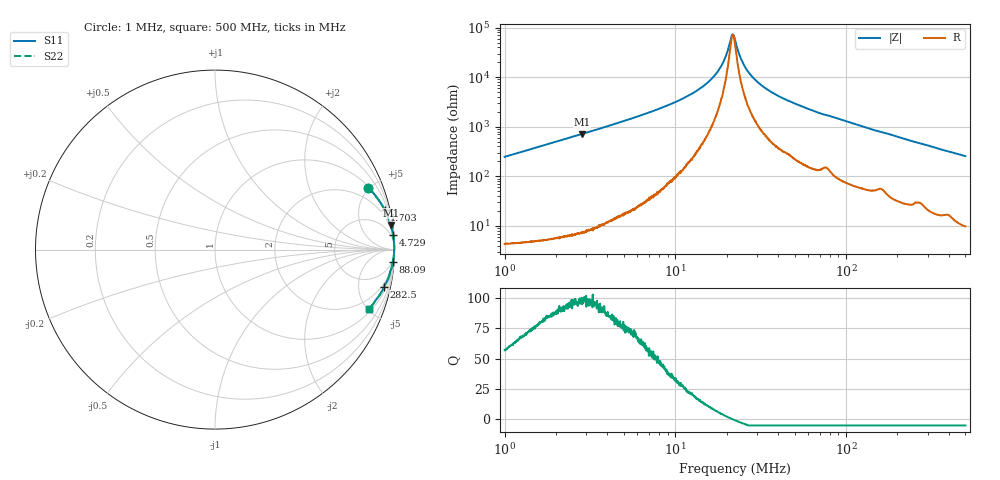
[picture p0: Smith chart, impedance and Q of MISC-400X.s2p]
!s-Parameter Generated by FASTRON Sdn. Bhd.
!FASTRON P/N : MISC-400X
!Keysight Technologies,E4991B,MY54100416,A.01.15
!Date: Thu Mar 26 11:04:12 2026
!Version  : Rev00 Thu Mar 26 11:04:12 2026
!Data & Calibration Information:
!PortZ  Port1:50+j0  Port2:50+j0
!When reading, reference impedance value at option line is always used.
!Remarks : This data is being provided solely for informational purposes.
!Freq	S11	S21	S12	S22
# Hz S dB R 50
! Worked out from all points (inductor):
!   1601 points, 1 MHz to 500 MHz, reference 50 ohm
!   read as one part in series: L = 39.3 uH near 1.032 MHz
!   highest Q = 97.7 at 2.843 MHz (marker M1), where L = 40 uH
!   self-resonance near 21.68 MHz
!   S11 on the Smith chart (normalised r, x): 1 MHz: 1.09, +4.95; 1.703 MHz: 1.10, +8.45; 4.729 MHz: 1, +25; 88.09 MHz: 3, -30; 282.5 MHz: 1.52, -8.95; 500 MHz: 1.20, -5.10
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1000000  -0.71 21.9  -8.57 -67.1  -8.57 -67.1  -0.71 21.9
1702548  -0.26 13.3  -12.78 -76.0  -12.78 -76.0  -0.26 13.3
2820919  -0.10 8.0  -17.10 -81.4  -17.10 -81.4  -0.10 8.0
2842918  -0.10 8.0  -17.17 -81.4  -17.17 -81.4  -0.10 8.0
4728708  -0.04 4.7  -21.81 -84.6  -21.81 -84.6  -0.04 4.7
7957584  -0.02 2.5  -27.16 -86.3  -27.16 -86.3  -0.02 2.5
1.178023e7  -0.01 1.4  -32.35 -86.1  -32.35 -86.1  -0.01 1.4
1.552103e7  -0.01 0.7  -37.93 -84.1  -37.93 -84.1  -0.01 0.7
1.870207e7  -0.01 0.3  -44.84 -77.1  -44.84 -77.1  -0.01 0.3
1.97472e7  -0.01 0.2  -48.48 -69.3  -48.48 -69.3  -0.01 0.2
2.142543e7  -0.01 0.0  -56.98 -20.8  -56.98 -20.8  -0.01 0.0
2.193061e7  -0.01 -0.0  -56.67 13.1  -56.67 13.1  -0.01 -0.0
2.236068e7  -0.01 -0.1  -55.23 35.5  -55.23 35.5  -0.01 -0.1
2.370216e7  -0.01 -0.2  -49.12 66.1  -49.12 66.1  -0.01 -0.2
2.522189e7  -0.01 -0.3  -44.91 74.3  -44.91 74.3  -0.01 -0.3
3.015594e7  -0.02 -0.7  -38.19 81.4  -38.19 81.4  -0.02 -0.7
4.066875e7  -0.02 -1.4  -32.24 83.5  -32.24 83.5  -0.02 -1.4
6.307767e7  -0.04 -2.6  -26.68 83.5  -26.68 83.5  -0.04 -2.6
8.809378e7  -0.06 -3.8  -23.48 82.5  -23.48 82.5  -0.06 -3.8
1.77937e8  -0.15 -7.9  -17.21 78.9  -17.21 78.9  -0.15 -7.9
2.824894e8  -0.32 -12.4  -13.35 74.3  -13.35 74.3  -0.32 -12.4
5e8  -0.73 -21.1  -8.87 66.7  -8.87 66.7  -0.73 -21.1
